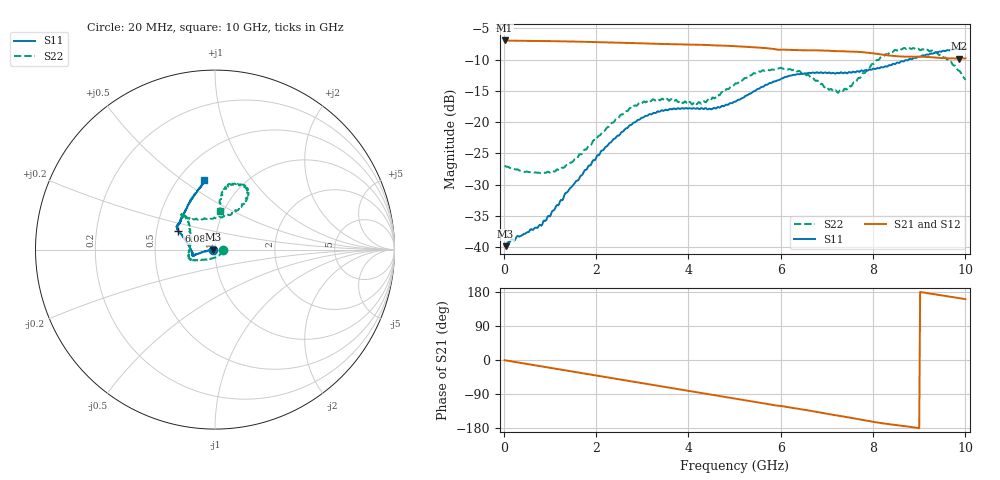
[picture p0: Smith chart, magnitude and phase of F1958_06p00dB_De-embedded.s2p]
! Integrated Device Technology
! Corporate Headquarters
! 6024 Silver Creek Valley Road
! San Jose, CA 95138  USA
! Phone:  1-408-284-8200
! Toll Free:  1-800-223-1366
! Webpage:  http://www.idt.com/
! Timing and RF Division
! 515 Groton Road, Suite 102
! Westford, MA 01886-6024
! Device:  F1958
! Description: 7-bit 0.25 dB Digital Step Attenuator
! Frequency:  0.001 -  6.000 GHz
! Package:  4x4 mm Thin QFN Plastic Package: 24 pin
! Ports:  2 RF, 12 DC
!  Pin  1  = D0
!  Pin  2  = VDD
!  Pin  3  = VMODE
!  Pin  4  = GND
!  Pin  5  = RF1  =  Port 1
!  Pin  6  = GND
!  Pin  7  = GND
!  Pin  8  = GND
!  Pin  9  = GND
!  Pin 10  = GND
!  Pin 11  = GND
!  Pin 12  = GND
!  Pin 13  = GND
!  Pin 14  = RF2  =  Port 2
!  Pin 15  = GND
!  Pin 16  = LE
!  Pin 17  = CLK
!  Pin 18  = DATA
!  Pin 19  = D6
!  Pin 20  = D5
!  Pin 21  = D4
!  Pin 22  = D3
!  Pin 23  = D2
!  Pin 24  = D1
! State:  24
! Atten State:  6.00 dB
! Voltage:  +3.30 Volts
! Current:  0.257 mA
! Data:  The device was measured on a F1958 evaluation board which has
!  individual transmission lines to the RF pins.  Data was collected
!  using a calibrated network analyzer.  The evaluation board was
!  de-embedded using Automatic Fixture Removal (AFR).
!  The reference plane is the edge of the package pin.
! Misc:
!  Action Tracker AT0419
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# GHz S dB R 50
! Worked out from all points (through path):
!   500 points, 20 MHz to 10 GHz, reference 50 ohm
!   highest |S21| = -6.93 dB at 20 MHz (marker M1); lowest = -9.8 dB at 9.86 GHz (marker M2)
!   group delay of S21, straight-line fit = 55.7 ps
!   lowest |S11| = -39.8 dB at 40 MHz (marker M3), VSWR 1.02, Z = 49 - j0.102 ohm
!   |S11| at or under -10 dB: start of sweep to 8.771 GHz
!   |S22| runs from -28.1 to -8.1 dB; largest |S21 - S12| = 0.0013
!   S11 on the Smith chart (normalised r, x): 20 MHz: 0.98, -0.00; 6.08 GHz: 0.65, +0.14; 10 GHz: 0.66, +0.61
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0.02  -39.75 -175.0  -6.93 -0.6  -6.93 -0.5  -26.93 -3.6
0.04  -39.85 -174.1  -6.94 -1.0  -6.93 -1.0  -27.07 -5.4
0.78  -36.43 -179.9  -7.01 -16.0  -7.01 -16.0  -28.12 -44.3
0.98  -35.02 -175.4  -7.03 -20.1  -7.03 -20.1  -28.03 -59.0
1.34  -31.33 -171.6  -7.07 -27.5  -7.07 -27.5  -27.01 -89.8
1.7  -28.46 -170.0  -7.13 -34.7  -7.13 -34.7  -25.02 -115.9
2.64  -21.03 -166.3  -7.31 -53.8  -7.30 -53.8  -18.24 -150.4
3.36  -18.32 -164.3  -7.48 -68.3  -7.48 -68.4  -16.41 -161.0
4.26  -17.85 -169.1  -7.63 -86.4  -7.64 -86.4  -16.97 167.4
5.02  -16.73 172.2  -7.84 -101.9  -7.85 -101.9  -13.80 136.0
5.52  -14.67 160.2  -8.07 -112.1  -8.08 -112.1  -11.88 131.7
6.08  -12.83 153.2  -8.40 -122.7  -8.42 -122.7  -11.43 133.3
6.68  -12.09 148.6  -8.51 -134.7  -8.53 -134.6  -12.89 128.8
7.08  -12.17 145.7  -8.59 -143.5  -8.60 -143.4  -14.69 108.6
7.3  -12.04 143.6  -8.64 -147.9  -8.64 -147.8  -14.97 90.9
7.9  -11.65 132.9  -8.90 -160.9  -8.89 -160.9  -11.36 60.7
8.34  -10.92 123.1  -9.33 -169.3  -9.33 -169.4  -9.02 58.5
8.76  -10.08 113.2  -9.53 -175.8  -9.54 -175.8  -8.09 64.7
9.26  -9.00 104.4  -9.63 174.7  -9.63 174.7  -8.54 76.5
9.54  -8.58 101.1  -9.74 169.5  -9.76 169.5  -9.69 81.1
9.86  -8.23 98.9  -9.83 163.5  -9.86 163.6  -11.77 83.2
10  -8.12 99.0  -9.79 160.5  -9.82 160.6  -13.24 82.6
